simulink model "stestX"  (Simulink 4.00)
settings: Solver=ode45  StartTime=0.0  StopTime=10.0  RelTol=1e-3

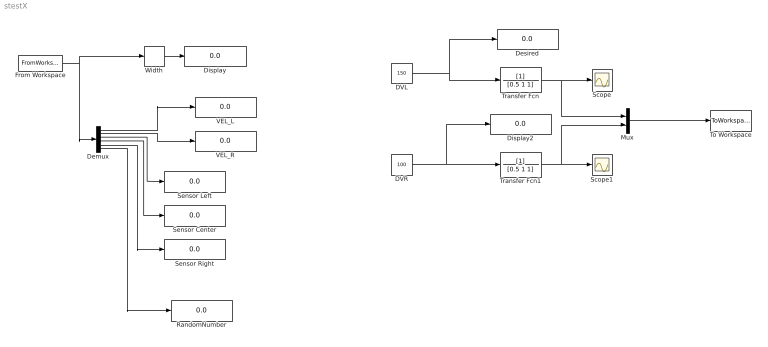
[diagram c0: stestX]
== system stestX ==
  DVL : Constant  Value=150
  DVR : Constant  Value=100
  Demux : Demux  Outputs=6  BusSelectionMode=off
  Desired : Display
  Display : Display
  Display2 : Display
  From Workspace : FromWorkspace  VariableName=data  SampleTime=0  OutputAfterFinalValue=Extrapolation
  Mux : Mux  Inputs=2
  RandomNumber : Display
  Scope : Scope
  Scope1 : Scope
  Sensor Center : Display
  Sensor Left : Display
  Sensor Right : Display
  To Workspace : ToWorkspace  VariableName=simout  SampleTime=-1  SaveFormat=Structure
  Transfer Fcn : TransferFcn  Numerator=[1]  Denominator=[0.5 1 1]  AbsoluteTolerance=auto  Realization=auto
  Transfer Fcn1 : TransferFcn  Numerator=[1]  Denominator=[0.5 1 1]  AbsoluteTolerance=auto  Realization=auto
  VEL_L : Display
  VEL_R : Display
  Width : Width
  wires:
  Width/1 -> Display/1
  From Workspace/1 -> Width/1, Demux/1
  Transfer Fcn/1 -> Scope/1, Mux/1
  Transfer Fcn1/1 -> Scope1/1, Mux/2
  Mux/1 -> To Workspace/1
  Demux/3 -> Sensor Left/1
  Demux/4 -> Sensor Center/1
  Demux/5 -> Sensor Right/1
  Demux/1 -> VEL_L/1
  Demux/2 -> VEL_R/1
  DVL/1 -> Transfer Fcn/1, Desired/1
  DVR/1 -> Transfer Fcn1/1, Display2/1
  Demux/6 -> RandomNumber/1
